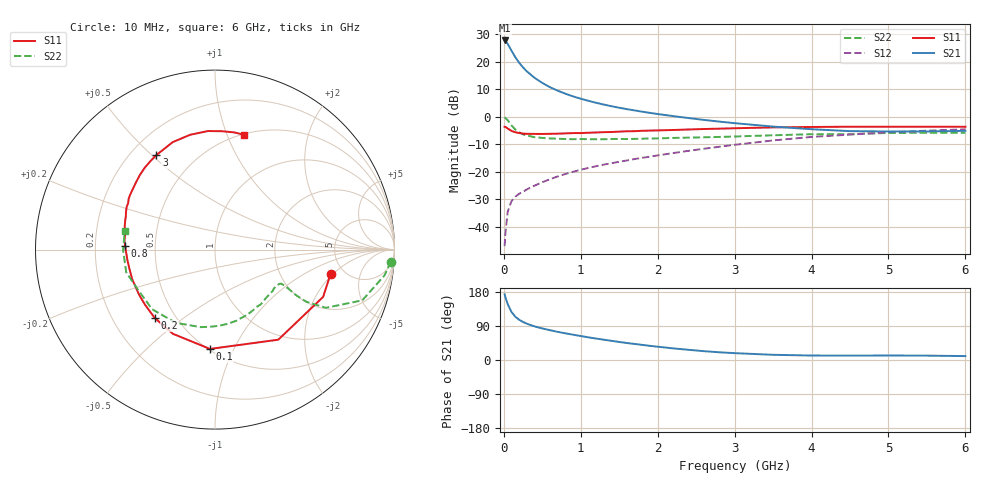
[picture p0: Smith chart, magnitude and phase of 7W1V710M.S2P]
! Infineon Technologies  Discrete & RF Semiconductors
! BFS17W
! Si NPN RF Bipolar Junction Transistor in SOT323
! VCE = 1.75 V  IC = 10 mA
! Common Emitter S-Parameters:  August  1999
# GHz  S  MA  R  50
!  f  S11  S21  S12  S22
! GHz  MAG  ANG  MAG  ANG  MAG  ANG  MAG  ANG
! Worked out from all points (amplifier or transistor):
!   36 points, 10 MHz to 6 GHz, reference 50 ohm
!   highest |S21| = 27.7 dB at 10 MHz (marker M1)
!   |S21| within 3 dB of that: start of sweep to 85.26 MHz
!   unconditionally stable (mu >= 1): 372.4 MHz to 3.161 GHz; 3.866 GHz to end of sweep
!   at 250 MHz: K = 0.83, MSG = 22.5 dB, |S12| = -27.2 dB
!   at 1.4 GHz: K = 1.25, MAG = 7.3 dB, |S12| = -16.8 dB
!   at 6 GHz: K = 1.09, MAG = -2.1 dB, |S12| = -4.5 dB
!   S11 on the Smith chart (normalised r, x): 10 MHz: 3.92, -1.86; 100 MHz: 0.51, -0.81; 200 MHz: 0.38, -0.39; 800 MHz: 0.33, +0.02; 3 GHz: 0.30, +0.52; 6 GHz: 0.51, +1.15
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0.01  0.6582 -11.8  24.3 173.4  0.0045 82.5  0.9822 -3.9
0.02  0.6576 -23.6  23.94 165.9  0.0076 80.3  0.9557 -8.6
0.05  0.6135 -54.9  21.09 147.4  0.0189 68.3  0.8681 -19.0
0.1  0.5541 -92.9  15.8 126.7  0.0296 54.6  0.6979 -27.7
0.15  0.5245 -116.6  12.01 114.1  0.0356 50.4  0.5868 -29.7
0.2  0.5077 -131.4  9.562 106.1  0.0402 51.8  0.5223 -29.4
0.25  0.4964 -141.9  7.857 100.3  0.0437 51.6  0.4808 -28.5
0.3  0.4918 -149.5  6.66 95.7  0.0483 53.7  0.458 -27.9
0.4  0.49 -160.5  5.092 88.7  0.0565 56.0  0.4272 -27.3
0.5  0.4887 -167.8  4.116 83.3  0.0651 58.4  0.4146 -27.2
0.6  0.4916 -173.4  3.446 78.6  0.0737 59.8  0.4059 -28.1
0.7  0.4952 -178.0  2.982 74.3  0.0829 61.2  0.4 -29.7
0.8  0.5004 177.8  2.628 70.4  0.0918 62.1  0.3958 -31.6
1.1  0.5146 167.9  1.949 59.7  0.1183 63.6  0.3928 -38.7
1.3  0.5267 161.7  1.668 53.5  0.136 63.9  0.392 -44.5
1.6  0.5465 154.2  1.377 44.8  0.1616 64.1  0.395 -53.5
2.2  0.5767 140.1  1.031 30.7  0.2199 63.8  0.4138 -73.4
3  0.6197 121.8  0.767 18.1  0.3106 59.6  0.4395 -100.7
3.5  0.6434 111.5  0.665 13.7  0.3733 55.0  0.4627 -118.2
4.5  0.6617 93.4  0.55 11.5  0.4763 42.5  0.4836 -152.2
5.5  0.6617 80.7  0.542 11.5  0.5602 30.7  0.512 -179.7
6  0.6597 75.8  0.557 10.3  0.5937 24.9  0.5138 168.1
